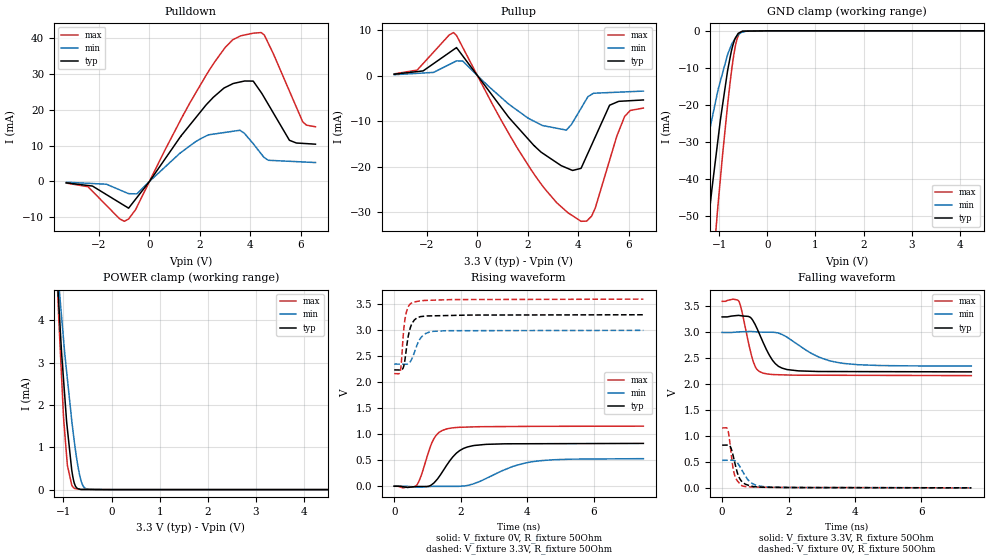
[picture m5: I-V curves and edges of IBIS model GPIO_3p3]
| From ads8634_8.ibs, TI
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|   GPIO_3p3   3.3V digital input Model
[Model] GPIO_3p3  | 3.3V digital input
Model_type I/O
Vinl = 0.99
Vinh = 2.31
Polarity   Non-Inverting
Vmeas = 1.65
Vref = 1.65
Cref = 15pF
Rref = 50
|   typ   min   max
|   (nom PVT)   (Fast PVT)   (slow PVT)
|BUFFER as INPUT
|C_comp from L-C Tank method(L=1nH)
|Resonant Frequency(Hz)   4.07G   4.63G   4.04G
|C_comp   1.52785E-12  1.18058E-12  1.55626E-12
|BUFFER OUTPUT TURNED HIGH
|C_comp from L-C Tank method(L=1nH)
|Resonant Frequency(Hz)   4.25G   4.93G   4.21G
|C_comp   1.40631E-12   1.04251E-12   1.43245E-12
|BUFFER OUTPUT TURNED LOW
|C_comp from L-C Tank method(L=1nH)
|Resonant Frequency(Hz)   4.38G   5.00G   4.25G
C_comp   1.32472E-12   1.01282E-12   1.40631E-12
| Where   nom PVT is  Nominal Process, 3.3V, 25C
|   Fast PVT is Strong Process, 3.6V, -40C
|   Slow PVT is Weak Process, 3.0V, 85C
|C_comp - from L-C Tank method, L = 1nH, peak frequency
[Model Spec]   | 3.3V
Vinl   0.99   0.9   1.08
Vinh   2.31   2.1   2.52
|Vinl = 0.3 DVDD
|Vinh = 0.7 DVDD
[Voltage Range]   3.3   3   3.6
[Temperature Range]   27   125   -40
[Pullup Reference]   3.3   3   3.6
[Pulldown Reference]   0   0   0
[Power Clamp Reference]   3.3   3   3.6
[GND Clamp Reference]   0   0   0
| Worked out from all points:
|   slope of the pulldown table from 0 to 0.495 V, typ, clamps not added: 98.5 ohm
|   slope of the pullup table from 0 to 0.495 V, typ, clamps not added: 136 ohm
|   GND clamp passes 1 mA (typ) near -0.62 V on its own axis
|   POWER clamp passes 1 mA (typ) near -0.88 V on its own axis
|   falling waveform, V_fixture 3.3V, R_fixture 50Ohm: 20-80 % time 490ps typ, 1.06ns min, 304ps max; typ from 3.3 V to 2.24 V
|   rising waveform, V_fixture 0V, R_fixture 50Ohm: 20-80 % time 586ps typ, 1.19ns min, 379ps max; typ from 0.002 V to 0.825 V
|   rising waveform, V_fixture 3.3V, R_fixture 50Ohm: 20-80 % time 178ps typ, 265ps min, 130ps max; typ from 2.24 V to 3.3 V
|   falling waveform, V_fixture 0V, R_fixture 50Ohm: 20-80 % time 226ps typ, 337ps min, 162ps max; typ from 0.825 V to 0.002 V
[Pulldown]
|   Voltage   I(typ)   I(min)   I(max)
-3.3V     -387.3uA   -203.7uA   -451.8uA
-2.443V   -1.121mA   -505.1uA   -1.445mA
-1.18V    -5.929mA   -2.342mA   -10.44mA
-825.7mV  -7.436mA   -3.4mA     -10.47mA
-499.9mV  -4.512mA   -3.47mA    -7.147mA
2.246V    21.33mA    12.67mA    29.59mA
3.623V    27.8mA     14.13mA    40.65mA
4.112V    28.01mA    10.61mA    41.37mA
4.558V    23.42mA    6.669mA    40.88mA
5.56V     11.49mA    5.631mA    25.19mA
6.085V    10.63mA    5.452mA    16.66mA
6.59V     10.41mA    5.281mA    15.26mA
[GND Clamp]
|   Voltage   I(typ)   I(min)   I(max)
-3.3V     -333.7mA   -218.9mA   -423.9mA
-1.588V   -96.13mA   -55.21mA   -138mA
-1.503V   -85.33mA   -48.26mA   -123.8mA
-1.25V    -54.2mA    -29.86mA   -82.26mA
-1.15V    -42.44mA   -23.67mA   -66.51mA
-1.037V   -30.42mA   -16.64mA   -48.59mA
-827.1mV  -10.74mA   -6.403mA   -20.01mA
-751.5mV  -5.648mA   -3.916mA   -11.52mA
-698.7mV  -3.133mA   -2.674mA   -6.534mA
-629.4mV  -1.185mA   -1.374mA   -2.162mA
-518.2mV  -90.78uA   -363.5uA   -142.2uA
6.59V     0A         0A         0A
[Pullup]
|   Voltage   I(typ)   I(min)   I(max)
-3.3V     282.6uA    176.8uA    359.8uA
-2.384V   863.4uA    472.1uA    1.213mA
-946.2mV  5.668mA    2.885mA    9.425mA
-576.3mV  4.273mA    3.16mA     6.132mA
1.319V    -9.636mA   -6.582mA   -13.42mA
2.588V    -17.04mA   -10.98mA   -24.23mA
3.533V    -20.27mA   -11.98mA   -29.82mA
4.119V    -20.33mA   -7.18mA    -32mA
4.537V    -15.25mA   -4.151mA   -30.86mA
5.249V    -6.525mA   -3.741mA   -18.61mA
5.848V    -5.597mA   -3.6mA     -8.981mA
6.59V     -5.369mA   -3.424mA   -7.142mA
[POWER Clamp]
|   Voltage   I(typ)   I(min)   I(max)
-3.3V     58.05mA    46.12mA    73.37mA
-1.159V   5.65mA     5.888mA    5.789mA
-1.098V   4.421mA    4.917mA    4.057mA
-1.077V   3.993mA    4.59mA     3.555mA
-1.002V   2.669mA    3.61mA     1.806mA
-918.3mV  1.436mA    2.622mA    575uA
-827.1mV  458.1uA    1.631mA    107.4uA
-762.1mV  114.7uA    1.036mA    23.91uA
-705.1mV  24.12uA    592.4uA    14.48uA
-628.4mV  4.506uA    187.8uA    2.951uA
-510.7mV  3.641uA    10.95uA    2.388uA
6.59V     0A         0A         0A
[Ramp]
R_load = 50
|   typ   min   max
dV/dt_r   0.493895/5.82202e-010  0.318267/1.16641e-009  0.693599/3.77544e-010
dV/dt_f   0.636389/4.88606e-010  0.388684/1.04633e-009  0.860088/3.02755e-010
[Falling Waveform]
V_fixture = 3.3V
V_fixture_min = 3V
V_fixture_max = 3.6V
R_fixture = 50Ohm
C_fixture = 0F
|   Time   V(typ)   V(min)   V(max)
0s        3.299V     2.999V     3.6V
503.7ps   3.328V     3.01V      3.602V
938.1ps   3.217V     3.015V     2.437V
1.051ns   3.074V     3.01V      2.285V
1.23ns    2.813V     3.005V     2.215V
1.601ns   2.398V     2.998V     2.185V
1.96ns    2.283V     2.905V     2.179V
2.849ns   2.247V     2.543V     2.174V
3.627ns   2.245V     2.404V     2.173V
7.5ns     2.238V     2.351V     2.166V
[Rising Waveform]
V_fixture = 0V
V_fixture_min = 0V
V_fixture_max = 0V
R_fixture = 50Ohm
C_fixture = 0F
|   Time   V(typ)   V(min)   V(max)
0s        1.562mV    1.115mV    647.2uV
666.3ps   -4.034mV   -13.4mV    14.25mV
796.7ps   -3.874mV   -14.65mV   179.1mV
1.185ns   58.23mV    -1.457mV   905.1mV
1.355ns   187.5mV    -1.368mV   1.039V
1.589ns   413.3mV    -1.246mV   1.105V
1.974ns   687.9mV    -692.5uV   1.135V
2.41ns    785.2mV    52.91mV    1.143V
4.131ns   818.6mV    470.3mV    1.152V
7.5ns     824.7mV    531.6mV    1.157V
[Rising Waveform]
V_fixture = 3.3V
V_fixture_min = 3V
V_fixture_max = 3.6V
R_fixture = 50Ohm
C_fixture = 0F
|   Time   V(typ)   V(min)   V(max)
0s        2.238V     2.351V     2.166V
183.1ps   2.237V     2.349V     2.206V
268.5ps   2.274V     2.348V     2.874V
326.2ps   2.444V     2.348V     3.218V
385.6ps   2.737V     2.351V     3.391V
489.2ps   3.058V     2.403V     3.51V
581.6ps   3.176V     2.528V     3.543V
807.1ps   3.265V     2.862V     3.568V
1.182ns   3.279V     2.981V     3.58V
7.5ns     3.299V     2.999V     3.6V
[Falling Waveform]
|Gnd
V_fixture = 0V
V_fixture_min = 0V
V_fixture_max = 0V
R_fixture = 50Ohm
C_fixture = 0F
|   Time   V(typ)   V(min)   V(max)
0s        824.8mV    532.1mV    1.157V
168ps     826.4mV    533.2mV    1.126V
254.2ps   787.6mV    533.8mV    762.8mV
316.7ps   661mV      534.2mV    433.9mV
369.3ps   520mV      529.5mV    265.3mV
483.2ps   245.2mV    461.9mV    117.1mV
643.7ps   94.48mV    288.3mV    31.65mV
902.8ps   31.56mV    86.38mV    17.95mV
1.239ns   12.19mV    24.67mV    13.96mV
7.5ns     1.614mV    1.435mV    647.8uV
